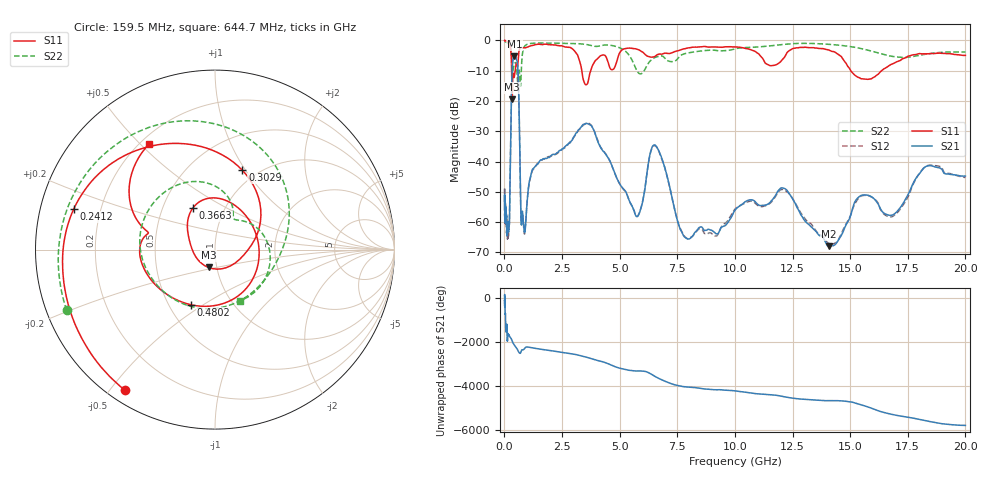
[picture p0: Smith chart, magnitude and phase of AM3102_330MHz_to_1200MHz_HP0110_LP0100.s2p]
! Date/Time: Tue, Sep 11, 2018 5:14 PM
! Network Analyzer: Agilent Technologies E8362B Rev: A.07.50.63
! Sweep from 0.010 to 20.000 GHz, 1601 Points, Sweep Type: LOG
! Power Supply: 4.949 V, 0.001 A
# Hz S DB R 50
!freq MagS11 AngS11 MagS21 AngS21 MagS12 AngS12 MagS22 AngS22
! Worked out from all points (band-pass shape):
!   1601 points, 10 MHz to 20 GHz, reference 50 ohm
!   highest |S21| = -5.26 dB at 432.6 MHz (marker M1); lowest = -67.9 dB at 14.07 GHz (marker M2)
!   |S21| within 3 dB of the highest: 345.2 MHz to 576.4 MHz (231.1 MHz wide, 50.2 % of centre)
!   lowest |S11| = -19.5 dB at 337.9 MHz (marker M3), VSWR 1.24, Z = 45.6 - j9.2 ohm
!   |S11| at or under -10 dB: 314.9 MHz to 470.2 MHz (155.4 MHz wide, 39.6 % of centre); 3.359 GHz to 3.746 GHz (387.2 MHz wide, 10.9 % of centre); 15.03 GHz to 16.37 GHz (1.342 GHz wide, 8.55 % of centre)
!   |S22| runs from -15.1 to -0.2 dB; largest |S21 - S12| = 0.0087
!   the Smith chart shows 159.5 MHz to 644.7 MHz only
!   S11 on the Smith chart (normalised r, x): 159.5 MHz: 0.05, -0.55; 241.2 MHz: 0.10, +0.14; 302.9 MHz: 0.85, +0.97; 366.3 MHz: 0.71, +0.35; 480.2 MHz: 0.64, -0.45; 644.7 MHz: 0.23, +0.53
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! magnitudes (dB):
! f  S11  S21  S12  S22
! 10 MHz  0.0  -51.3  -57.2  -0.2
! 35.55 MHz  0.0  -59.2  -60.4  -0.4
! 126.4 MHz  -0.4  -62.1  -64.2  -0.8
! 159.5 MHz  -0.6  -62.2  -64.3  -1.0
! 241.2 MHz  -1.7  -49.6  -49.9  -1.8
! 302.9 MHz  -6.6  -19.9  -19.9  -4.2
! 337.9 MHz  -19.5  -9.3  -9.4  -8.4
! 366.3 MHz  -11.6  -6.6  -6.7  -10.0
! 432.6 MHz  -11.9  -5.3  -5.3  -7.9
! 447.2 MHz  -11.2  -5.3  -5.3  -7.6
! 480.2 MHz  -9.5  -5.5  -5.5  -7.3
! 644.7 MHz  -3.2  -25.3  -25.4  -10.0
! 726 MHz  -2.3  -60.0  -59.6  -11.7
! 865.5 MHz  -2.4  -62.9  -63.8  -2.1
! 1.59 GHz  -1.4  -39.5  -39.5  -0.9
! 3.668 GHz  -12.2  -27.7  -27.4  -1.5
! 5.652 GHz  -2.7  -56.8  -56.8  -8.4
! 6.549 GHz  -5.2  -34.6  -34.8  -5.6
! 7.882 GHz  -2.6  -65.3  -65.2  -4.3
! 12.09 GHz  -6.1  -48.7  -49.2  -1.3
! 14.07 GHz  -3.2  -67.9  -67.0  -1.3
! 20 GHz  -5.0  -44.8  -45.3  -3.8
